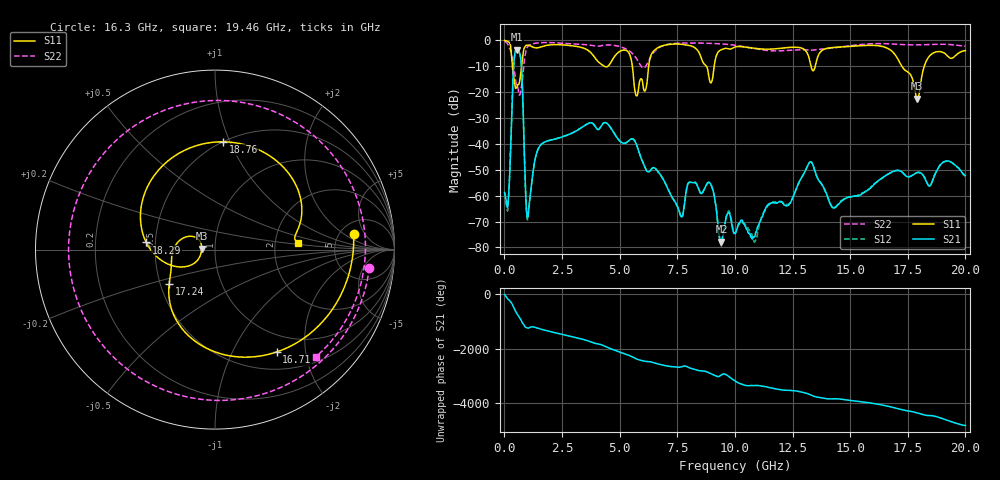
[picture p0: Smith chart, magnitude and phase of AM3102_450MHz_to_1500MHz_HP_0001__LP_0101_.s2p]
!Agilent Technologies,E8364B,MY43040894,A.07.50.67
!Agilent E8364B: A.07.50.67
!Date: Thursday, January 11, 2018 05:20:41
!Correction: S11(Full 2 Port(1,2))
!S21(Full 2 Port(1,2))
!S12(Full 2 Port(1,2))
!S22(Full 2 Port(1,2))
!S2P File: Measurements: S11, S21, S12, S22:
# Hz S  dB  R 50
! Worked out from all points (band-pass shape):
!   1601 points, 10 MHz to 20 GHz, reference 50 ohm
!   highest |S21| = -3.57 dB at 547.2 MHz (marker M1); lowest = -77.7 dB at 9.418 GHz (marker M2)
!   |S21| within 3 dB of the highest: 433.8 MHz to 701.2 MHz (267.4 MHz wide, 47.1 % of centre)
!   lowest |S11| = -22.6 dB at 17.91 GHz (marker M3), VSWR 1.16, Z = 43.1 + j0.407 ohm
!   |S11| at or under -10 dB: 348.6 MHz to 744.2 MHz (395.5 MHz wide, 72.4 % of centre); 5.552 GHz to 6.258 GHz (706 MHz wide, 12 % of centre); 17.24 GHz to 18.21 GHz (971.6 MHz wide, 5.48 % of centre)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
!   |S22| runs from -21.2 to -0.4 dB; largest |S21 - S12| = 0.0062
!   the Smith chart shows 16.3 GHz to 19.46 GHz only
!   S11 on the Smith chart (normalised r, x): 16.3 GHz: 6.60, +2.99; 16.71 GHz: 0.74, -1.51; 17.24 GHz: 0.56, -0.24; 18.29 GHz: 0.44, +0.04; 18.76 GHz: 0.50, +0.95; 19.46 GHz: 2.69, +0.24
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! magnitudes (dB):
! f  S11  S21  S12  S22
! 10 MHz  0.0  -58.7  -59.0  -0.4
! 547.2 MHz  -18.1  -3.6  -3.6  -17.9
! 722.1 MHz  -11.6  -8.1  -8.1  -18.9
! 1.022 GHz  -1.9  -68.3  -69.1  -2.3
! 1.534 GHz  -2.7  -40.9  -40.9  -0.9
! 3.346 GHz  -2.8  -33.7  -33.7  -1.6
! 5.732 GHz  -21.5  -40.3  -40.3  -7.0
! 6.682 GHz  -2.7  -50.9  -51.0  -3.0
! 8.918 GHz  -16.0  -55.0  -55.2  -1.2
! 9.418 GHz  -3.6  -77.7  -79.5  -1.4
! 10.01 GHz  -2.5  -74.7  -74.5  -1.9
! 13.34 GHz  -11.1  -47.3  -47.3  -3.8
! 14.29 GHz  -2.7  -64.7  -64.6  -2.9
! 16.3 GHz  -2.2  -53.7  -53.8  -1.3
! 16.68 GHz  -3.3  -51.5  -51.5  -1.3
! 16.71 GHz  -3.5  -51.3  -51.3  -1.4
! 17.24 GHz  -9.9  -50.8  -50.8  -1.6
! 17.91 GHz  -22.6  -51.0  -51.1  -1.8
! 18.29 GHz  -8.3  -54.2  -54.1  -1.7
! 18.76 GHz  -4.4  -50.3  -50.3  -1.5
! 19.46 GHz  -6.7  -47.6  -47.5  -1.7
! 20 GHz  -4.0  -52.1  -52.4  -2.3
